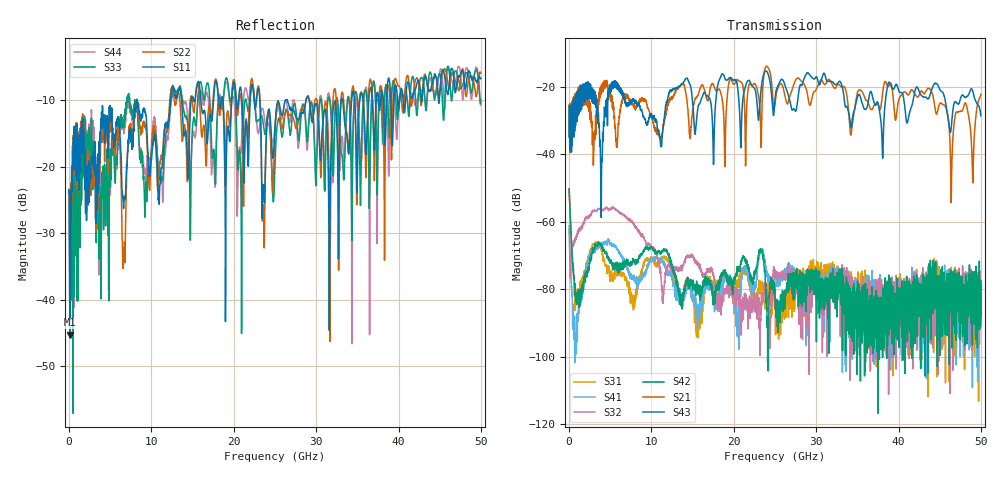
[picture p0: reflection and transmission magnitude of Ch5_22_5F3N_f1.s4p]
!Agilent Technologies,N5247A,US51170199,A.09.90.13
!Agilent N5247A: A.09.90.13
!Date: Wednesday, December 09, 2015 09:42:57
!Correction: S11(Full 4 Port(1,2,3,4))
!S12(Full 4 Port(1,2,3,4))
!S13(Full 4 Port(1,2,3,4))
!S14(Full 4 Port(1,2,3,4))
!S21(Full 4 Port(1,2,3,4))
!S22(Full 4 Port(1,2,3,4))
!S23(Full 4 Port(1,2,3,4))
!S24(Full 4 Port(1,2,3,4))
!S31(Full 4 Port(1,2,3,4))
!S32(Full 4 Port(1,2,3,4))
!S33(Full 4 Port(1,2,3,4))
!S34(Full 4 Port(1,2,3,4))
!S41(Full 4 Port(1,2,3,4))
!S42(Full 4 Port(1,2,3,4))
!S43(Full 4 Port(1,2,3,4))
!S44(Full 4 Port(1,2,3,4))
!S4P File: Measurements: <S11,S12,S13,S14>,
!<S21,S22,S23,S24>,
!<S31,S32,S33,S34>,
!<S41,S42,S43,S44>:
# Hz S  dB  R 50
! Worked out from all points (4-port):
!   3201 points, 10 MHz to 50 GHz, reference 50 ohm
!   strongest paths, dB at 10 MHz, 12.51 GHz, 25 GHz, 37.5 GHz, 50 GHz:
!     S43: -35.0, -21.2, -23.8, -24.7, -28.6
!     S21: -34.5, -23.5, -25.2, -25.1, -22.2
!     S42: -50.2, -73.1, -80.6, -116.8, -88.0
!     S32: -62.0, -73.8, -75.3, -87.3, -81.2
!     S41: -61.2, -76.7, -77.1, -84.1, -89.7
!     S31: -50.4, -75.0, -84.7, -84.6, -87.5
!   lowest |S11| = -45.3 dB at 88.11 MHz (marker M1), VSWR 1.01, Z = 50.3 + j0.471 ohm
!   |S11| at or under -10 dB: start of sweep to 8.22 GHz; 8.243 GHz to 12.29 GHz (4.047 GHz wide, 39.4 % of centre); 29.15 GHz to 33.05 GHz (3.902 GHz wide, 12.5 % of centre)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
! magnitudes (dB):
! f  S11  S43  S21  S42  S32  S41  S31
! 10 MHz  -23.8  -35.0  -34.5  -50.2  -62.0  -61.2  -50.4
! 88.11 MHz  -45.3  -38.4  -39.6  -54.4  -70.4  -66.3  -54.4
! 1.01 GHz  -17.8  -26.6  -22.9  -82.6  -63.7  -95.5  -82.1
! 3.931 GHz  -12.6  -48.5  -19.7  -67.3  -56.3  -66.4  -68.4
! 43.67 GHz  -8.6  -23.4  -20.4  -72.5  -81.2  -82.9  -81.9
! 46.42 GHz  -5.2  -31.6  -50.4  -81.8  -85.5  -92.0  -80.8
! 50 GHz  -6.7  -28.6  -22.2  -88.0  -81.2  -89.7  -87.5
